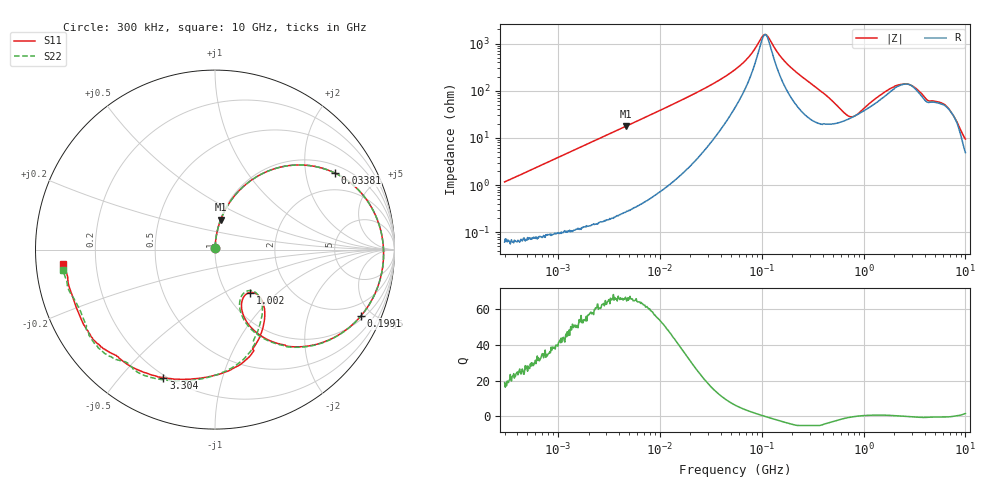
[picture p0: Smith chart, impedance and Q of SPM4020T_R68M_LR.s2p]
! S-Parameter Data Generated by TDK Corporation
! Copyright(C) 2024 TDK Corporation.
! All Rights Reserved.
! TDK P/N: SPM4020T-R68M-LR (SMD / SMT Inductor (Coil))
! Property: L=680nH at 100kHz
! Size(LxWxT): 4.4x4.1x2mm
! Model Type: s2p (Touchstone File Format Version 1.0)
! Frequency: DC=Yes Start=0.3MHz Stop=10000MHz 802points Log-sweep
! Model Generated on May 28, 2024
! Terms and conditions regarding TDK Simulation Models:
! 1)This simulation model is being provided solely for informational
!  purposes. Please refer to the specifications of the products in
!  terms of detailed characteristics of such products.
! 2)In no event shall TDK Corporation of any of its subsidiaries be
!  liable for any loss or damage arising, directly or indirectly,
!  from any information contained in this simulation model, including,
!  but not limited to loss or damages arising from any inaccuracies,
!  omissions or errors in connection with such information.
! 3)Any and all copyrights on this simulation model are owned by
!  TDK Corporation.  Duplication or redistribution of this simulation
!  model without prior written permission from TDK Corporation
!  is prohibited.
! 4)This simulation model is subject to any modification or change
!  without any prior notice.
! 5)Neither TDK Corporation nor any of its subsidiaries shall make any
!  warranty, express or implied, including but not limited to the
!  correctness, implied warranties of merchantability and fitness for
!  a particular purpose with respect to this simulation models.
! 6)The use of this simulation model shall be deemed to have consented
!  to the terms and conditions hereof.
! Port Assignments:
!  1 ---@@@--- 2
! Applicable Conditions:
!  Temperature = 25 degC
!  DC Bias Current = 0 A
!  Small Signal Operation
# Hz S MA R 50
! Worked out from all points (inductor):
!   801 points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, 300 kHz to 10 GHz, reference 50 ohm
!   read as one part in series: L = 612 nH near 318.3 kHz
!   highest Q = 66 at 4.611 MHz (marker M1), where L = 603 nH
!   self-resonance near 108.5 MHz
!   S11 on the Smith chart (normalised r, x): 300 kHz: 1.00, +0.02; 33.81 MHz: 1.27, +2.92; 199.1 MHz: 1.18, -4.31; 1.002 GHz: 1.28, -0.68; 3.304 GHz: 0.19, -0.66; 10 GHz: 0.08, -0.05
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300000  0.01165 86.2  0.9993 -0.7  0.9993 -0.7  0.01144 86.4
1713600  0.06433 85.1  0.9967 -3.8  0.9967 -3.8  0.06435 85.2
4611084  0.1702 79.2  0.9828 -10.0  0.9828 -10.0  0.1703 79.1
9671944  0.3408 68.7  0.9338 -20.3  0.9339 -20.3  0.3408 68.6
2.036513e7  0.6115 49.6  0.771 -38.5  0.7711 -38.5  0.6115 49.6
3.38066e7  0.7926 32.6  0.559 -53.6  0.5591 -53.6  0.7926 32.6
5.477226e7  0.8974 16.4  0.3223 -64.6  0.3223 -64.6  0.8975 16.4
7.329659e7  0.9276 7.5  0.1877 -65.1  0.1878 -65.1  0.9277 7.4
1.080141e8  0.9399 -4.1  0.06008 -5.7  0.0601 -5.8  0.9399 -4.2
1.990845e8  0.8932 -24.4  0.2945 52.9  0.2945 52.9  0.8931 -24.6
3.126428e8  0.7732 -43.1  0.5211 37.5  0.5212 37.5  0.7726 -43.4
4.269249e8  0.6313 -56.1  0.6529 21.8  0.653 21.8  0.63 -56.6
5.99416e8  0.4441 -66.2  0.7414 1.4  0.7414 1.4  0.4402 -67.2
7.726947e8  0.3315 -63.4  0.7467 -15.0  0.7468 -15.1  0.3228 -64.8
1.001841e9  0.3085 -50.8  0.6968 -32.3  0.6969 -32.3  0.2939 -51.3
1.323741e9  0.3929 -47.5  0.5856 -50.9  0.5857 -50.9  0.3745 -47.3
1.767019e9  0.526 -60.3  0.4198 -66.1  0.4198 -66.1  0.4905 -59.6
2.264206e9  0.6608 -78.9  0.3152 -70.4  0.3154 -70.5  0.6301 -75.2
3.303594e9  0.7685 -111.9  0.2344 -66.8  0.2344 -66.8  0.7661 -107.5
4.22443e9  0.8063 -130.0  0.2425 -73.9  0.2426 -74.0  0.8028 -126.1
6.333834e9  0.8422 -143.1  0.1911 -92.7  0.1911 -92.8  0.8502 -140.0
1e10  0.8493 -174.4  0.1411 -126.8  0.1412 -126.9  0.8533 -172.3
